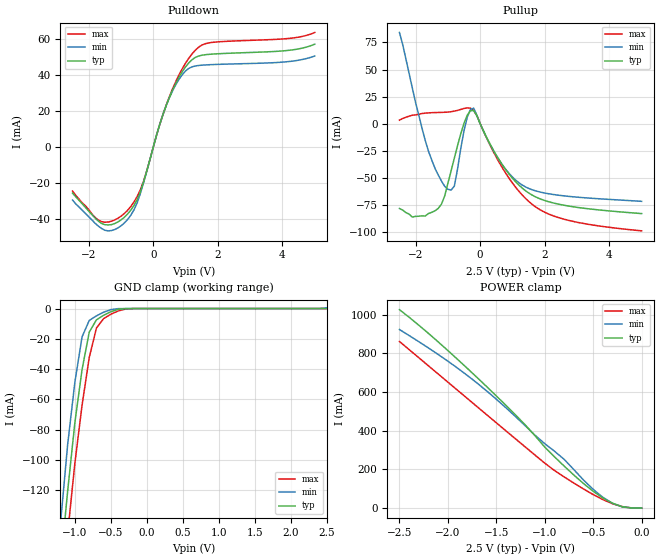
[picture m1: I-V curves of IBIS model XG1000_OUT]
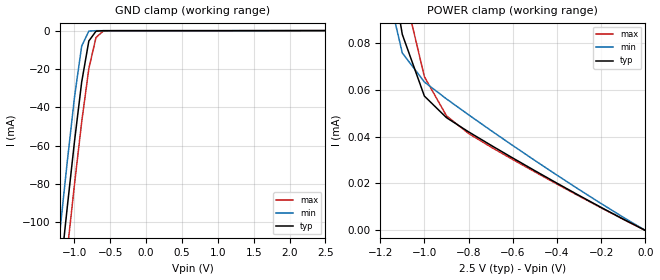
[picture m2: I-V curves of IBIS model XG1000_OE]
|   IBIS File xg1kca-d.ibs
|   Epson Toyocom Corporation , 2005
[IBIS Ver]   2.1
[Comment Char]   |_char
[File name]   xg1kca-d.ibs
[File Rev]   2.0
[Date]   2006/12/26
[Source]
[Notes]
[Disclaimer]
This information is for modeling purposes only, and is not guaranteed.
Property of Epson Toyocom Corp.,
unauthorized reproduction and/or distribution is strictly prohibited.
[Copyright]
Copyright 2002, Epson Toyocom Corp.
|   Component XG-1000CA_D
[Component]   XG-1000CA_D
[Manufacturer]   Epson Toyocom Corp.
[Package]
| variable   typ   min   max
R_pkg   0.878   NA   NA
L_pkg   2.13nH   NA   NA
C_pkg   3.21pF   NA   NA
[Pin]signal_name   model_name   R_pin   L_pin   C_pin
1   oe   XG1000_OE   NA   NA   NA
2   vss   GND   NA   NA   NA
3   out   XG1000_OUT   NA   NA   NA
4   vdd   POWER   NA   NA   NA
| Models and submodels in the file (2): XG1000_OUT (3-state), XG1000_OE (Input)
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|   Model XG1000_OUT
[Model]   XG1000_OUT
Model_type 3-state
Enable Active-High
Polarity Inverting
C_comp   3p   2.5p   3.5p
[Temperature Range] 25   -40   85
[Voltage Range]   2.5   2.35   2.65
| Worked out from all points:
|   slope of the pulldown table from 0 to 0.375 V, typ, clamps not added: 17.2 ohm
|   slope of the pullup table from 0 to 0.375 V, typ, clamps not added: 16.7 ohm
|   GND clamp passes 1 mA (typ) near -0.43 V on its own axis
|   POWER clamp passes 1 mA (typ) near -0.11 V on its own axis
[Pullup]
-2.5V     -78.2mA    84.14mA    3.272mA
-2.1V     -86.15mA   32.78mA    7.816mA
-1.6V     -82.82mA   -25.43mA   9.996mA
-1.2V     -74.31mA   -52.86mA   10.43mA
-1V       -55.08mA   -60.51mA   10.71mA
-800mV    -31.77mA   -57.59mA   11.59mA
-400mV    7.819mA    6.007mA    14.64mA
-200mV    12.11mA    14.3mA     12.12mA
700mV     -38.5mA    -38.5mA    -41.31mA
1.7V      -67.28mA   -61.81mA   -76.41mA
2.8V      -76.26mA   -67.2mA    -89.61mA
5V        -82.94mA   -71.63mA   -98.86mA
[Pulldown]
-2.5V     -25.69mA   -29.56mA   -24.57mA
-1.6V     -42.58mA   -45.4mA    -41.58mA
-1.2V     -42.67mA   -46.03mA   -40.69mA
-800mV    -37.42mA   -40.47mA   -35.35mA
-500mV    -29.28mA   -31.13mA   -27.61mA
-300mV    -19.42mA   -19.82mA   -19mA
400mV     23.13mA    23.1mA     23.31mA
800mV     39.05mA    37.82mA    40.32mA
1.1V      46.88mA    43.79mA    49.48mA
1.7V      51.58mA    45.81mA    57.93mA
4.1V      53.68mA    47.44mA    60.33mA
5V        57.29mA    50.7mA     63.79mA
[GND Clamp]
-2.5V     -829.1mA   -845.3mA   -829.6mA
-1.2V     -170.3mA   -142.5mA   -196.7mA
-1.1V     -120.7mA   -89.99mA   -148.9mA
-1V       -75.55mA   -48.78mA   -102.4mA
-900mV    -40.37mA   -18.72mA   -63.95mA
-800mV    -15.58mA   -7.854mA   -32.35mA
-700mV    -7.457mA   -4.83mA    -12.88mA
-600mV    -4.429mA   -2.41mA    -6.641mA
-500mV    -2.099mA   -692uA     -3.748mA
-400mV    -554.4uA   -62.41uA   -1.607mA
-300mV    -51.39uA   -1.685uA   -355.5uA
2.5V      3.498nA    506.5uA    -132.6nA
[POWER Clamp]
-2.5V     1.026A     923.1mA    861.3mA
-2.1V     859mA      793.9mA    693mA
-1.7V     675.5mA    646.7mA    524.7mA
-1.3V     480.6mA    472mA      356.9mA
-1V       315mA      332.7mA    231.9mA
-800mV    217mA      251.7mA    160.9mA
-600mV    126.5mA    144.8mA    98.33mA
-500mV    86.3mA     96.2mA     69.45mA
-400mV    51.62mA    55.26mA    43.48mA
-300mV    24.52mA    24.33mA    22.06mA
-200mV    6.958mA    5.264mA    7.215mA
0V        3.498nA    9.406pA    211.2nA
[Ramp]
R_load=50
dV/dt_r   1.103E+0/1.198E-10   1.042E+0/8.584E-11   1.190E+0/7.697E-11
dV/dt_f   1.076E+0/7.420E-11   1.011E+0/1.171E-10   1.145E+0/1.161E-10
|   Model XG1000_OE
[Model]   XG1000_OE
Model_type Input
Vinh=1.75
Vinl=0.75
C_comp   3p   2.5p   3.5p
[Temperature Range] 25   -40   85
[Voltage Range]   2.5   2.35   2.65
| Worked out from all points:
|   GND clamp passes 1 mA (typ) near -0.71 V on its own axis
|   POWER clamp passes 1 mA (typ) near -2.16 V on its own axis
[GND Clamp]
-2.5V     -614.1mA   -592.4mA   -635.3mA
-1.3V     -163.5mA   -139.8mA   -186.1mA
-1.2V     -127.3mA   -103.5mA   -150.1mA
-1.1V     -91.9mA    -68.14mA   -114.6mA
-1V       -57.88mA   -34.79mA   -80.24mA
-900mV    -26.95mA   -8.104mA   -47.82mA
-800mV    -5.421mA   -270.5uA   -19.87mA
-700mV    -321.6uA   -48.96uA   -3.606mA
-600mV    -52.31uA   -47.39uA   -322.8uA
2.5V      2.498pA    8.499uA    -6.762uA
[POWER Clamp]
-2.5V     1.329mA    1.311mA    1.351mA
-1.2V     139.2uA    116uA      167.8uA
-1.1V     83.49uA    75.59uA    105.3uA
-1V       57.21uA    63.22uA    65.47uA
-900mV    48.03uA    56.01uA    48.79uA
-800mV    41.98uA    49.25uA    41.29uA
-700mV    36.35uA    42.64uA    35.59uA
-300mV    14.9uA     17.42uA    14.64uA
0V        2.416pA    2.181pA    3.567pA
